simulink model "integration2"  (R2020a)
settings: Solver=ode45  StartTime=0.0  StopTime=4  RelTol=1e-3  EnableMultiTasking=on

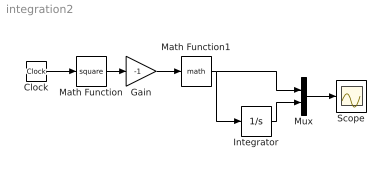
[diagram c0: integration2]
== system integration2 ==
  note: .
  Clock : Clock
  Gain : Gain  Gain=-1
  Integrator : Integrator
  Math Function : Math  Operator=square  SignedPower=on
  Math Function1 : Math  SignedPower=on
  Mux : Mux  Inputs=2
  Scope : Scope
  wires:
  Clock/1 -> Math Function/1
  Math Function/1 -> Gain/1
  Gain/1 -> Math Function1/1
  Math Function1/1 -> Integrator/1, Mux/1
  Mux/1 -> Scope/1
  Integrator/1 -> Mux/2
